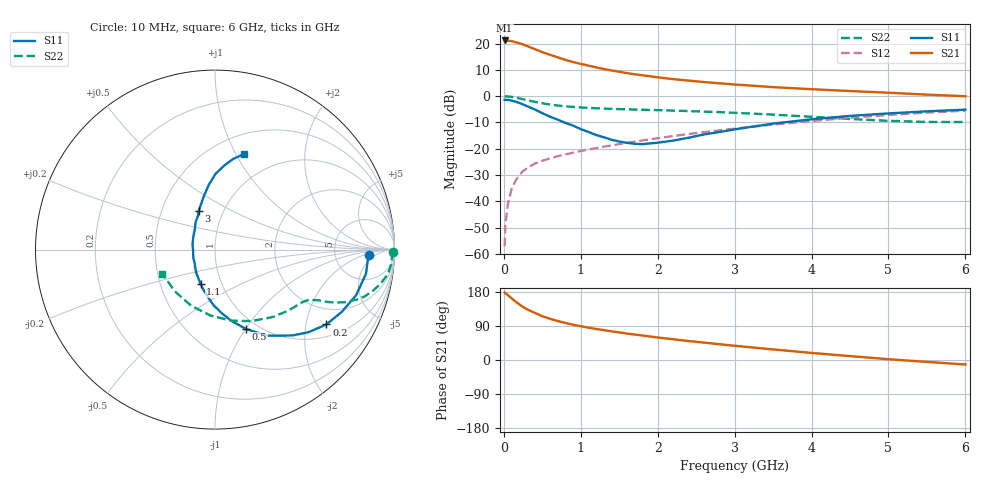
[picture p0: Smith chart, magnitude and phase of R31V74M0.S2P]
! SIEMENS Small Signal Semiconductors
! BFR181
! Si NPN RF Bipolar Junction Transistor in SOT23
! VCE = 1.75 V  IC = 4 mA
! Common Emitter S-Parameters:  May  1996
# GHz  S  MA  R  50
!  f  S11  S21  S12  S22
! GHz  MAG  ANG  MAG  ANG  MAG  ANG  MAG  ANG
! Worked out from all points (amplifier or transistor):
!   36 points, 10 MHz to 6 GHz, reference 50 ohm
!   highest |S21| = 21.2 dB at 10 MHz (marker M1)
!   |S21| within 3 dB of that: start of sweep to 377.3 MHz
!   unconditionally stable (mu >= 1): 1.167 GHz to 3.074 GHz
!   at 250 MHz: K = 0.37, MSG = 24.1 dB, |S12| = -28.5 dB
!   at 1.4 GHz: K = 1.05, MAG = 12.9 dB, |S12| = -18.7 dB
!   at 6 GHz: K = 0.86, MSG = 2.8 dB, |S12| = -5.5 dB
!   S11 on the Smith chart (normalised r, x): 10 MHz: 12, -3; 200 MHz: 1.39, -2.62; 500 MHz: 0.88, -1.00; 1.1 GHz: 0.79, -0.32; 3 GHz: 0.76, +0.35; 6 GHz: 0.70, +1.07
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0.01  0.8563 -2.0  11.49 178.2  0.0014 94.2  0.9935 -0.8
0.02  0.8536 -3.3  11.44 176.4  0.0035 85.3  0.9861 -1.7
0.05  0.8522 -9.0  11.34 171.4  0.0086 86.3  0.9877 -4.2
0.1  0.8264 -17.9  11.17 163.1  0.0169 82.0  0.9725 -8.1
0.15  0.7874 -26.1  10.66 154.3  0.0243 75.3  0.9405 -11.8
0.2  0.7476 -33.9  10.18 147.2  0.0313 72.2  0.9093 -14.6
0.25  0.6958 -41.4  9.659 140.0  0.0376 69.1  0.8749 -17.3
0.3  0.6455 -47.8  9.033 134.0  0.0428 67.1  0.8402 -19.3
0.4  0.561 -58.8  7.891 124.6  0.052 63.5  0.7819 -22.0
0.5  0.4743 -68.7  6.885 115.5  0.0591 61.4  0.7324 -23.8
0.6  0.4078 -77.0  6.133 108.7  0.0655 60.9  0.6926 -24.9
0.7  0.3572 -83.8  5.49 102.9  0.072 60.5  0.6637 -25.6
0.8  0.3106 -91.4  4.919 97.7  0.0779 59.9  0.6406 -26.1
0.9  0.2755 -97.0  4.468 93.1  0.0843 60.0  0.6249 -26.8
1.1  0.2088 -112.6  3.814 85.4  0.0964 60.8  0.5989 -28.0
1.6  0.1295 -158.7  2.748 69.8  0.1295 61.8  0.5624 -32.0
2.2  0.1427 147.2  2.112 54.7  0.1741 61.0  0.5321 -39.3
3  0.2335 113.0  1.67 37.5  0.2416 57.1  0.4827 -52.1
3.5  0.3008 102.2  1.487 27.9  0.2878 53.3  0.4462 -63.2
4.5  0.422 89.6  1.254 10.3  0.3879 43.2  0.3682 -93.8
5.5  0.5153 78.7  1.071 -5.0  0.4861 30.3  0.3229 -133.9
6  0.5548 73.3  0.998 -11.9  0.5298 23.2  0.3225 -155.6
